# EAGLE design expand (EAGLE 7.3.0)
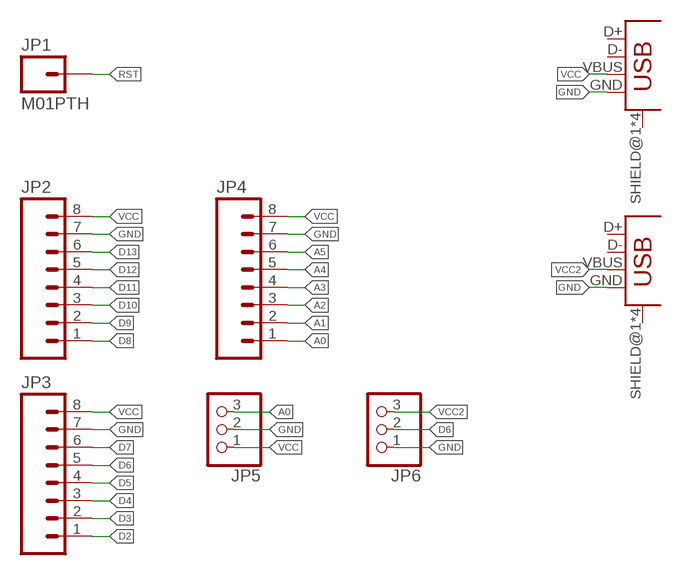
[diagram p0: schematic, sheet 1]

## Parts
JP1  M01PTH  [1X01]
JP2  M08  [1X08]
JP3  M08  [1X08]
JP4  M08  [1X08]
JP5  PINHD-1X3  [1X03]
JP6  PINHD-1X3  [1X03]
U$1  USB_MINIB  [USB_MINIB]
U$2  USB_MINIB  [USB_MINIB]

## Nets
A0: JP4.1 JP5.3
A1: JP4.2
A2: JP4.3
A3: JP4.4
A4: JP4.5
A5: JP4.6
D2: JP3.1
D3: JP3.2
D4: JP3.3
D5: JP3.4
D6: JP3.5 JP6.2
D7: JP3.6
D8: JP2.1
D9: JP2.2
D10: JP2.3
D11: JP2.4
D12: JP2.5
D13: JP2.6
GND: JP2.7 JP3.7 JP4.7 JP5.2 JP6.1 U$1.GND U$2.GND
RST: JP1.1
VCC: JP2.8 JP3.8 JP4.8 JP5.1 U$1.VBUS
VCC2: JP6.3 U$2.VBUS
Unconnected: U$1.D+ U$1.D- U$1.SHIELD@1(SHIELD) U$1.SHIELD@2(SHIELD) U$1.SHIELD@3(SHIELD) U$1.SHIELD@4(SHIELD) U$2.D+ U$2.D- U$2.SHIELD@1(SHIELD) U$2.SHIELD@2(SHIELD) U$2.SHIELD@3(SHIELD) U$2.SHIELD@4(SHIELD)

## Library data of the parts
JP1 = 01_SparkFun:M01: Header 1
JP2-JP4 = 01_SparkFun:M08: Header 8 Standard 8-pin 0.1" header. Use with straight break away headers (SKU : PRT-00116), right angle break away headers (PRT-00553), swiss pins (PRT-00743), machine pins (PRT-00117), and female headers (PRT-00115).
JP5 JP6 = adafruit:PINHD-1X3: PIN HEADER
U$1 U$2 = fab:USB_MINIB

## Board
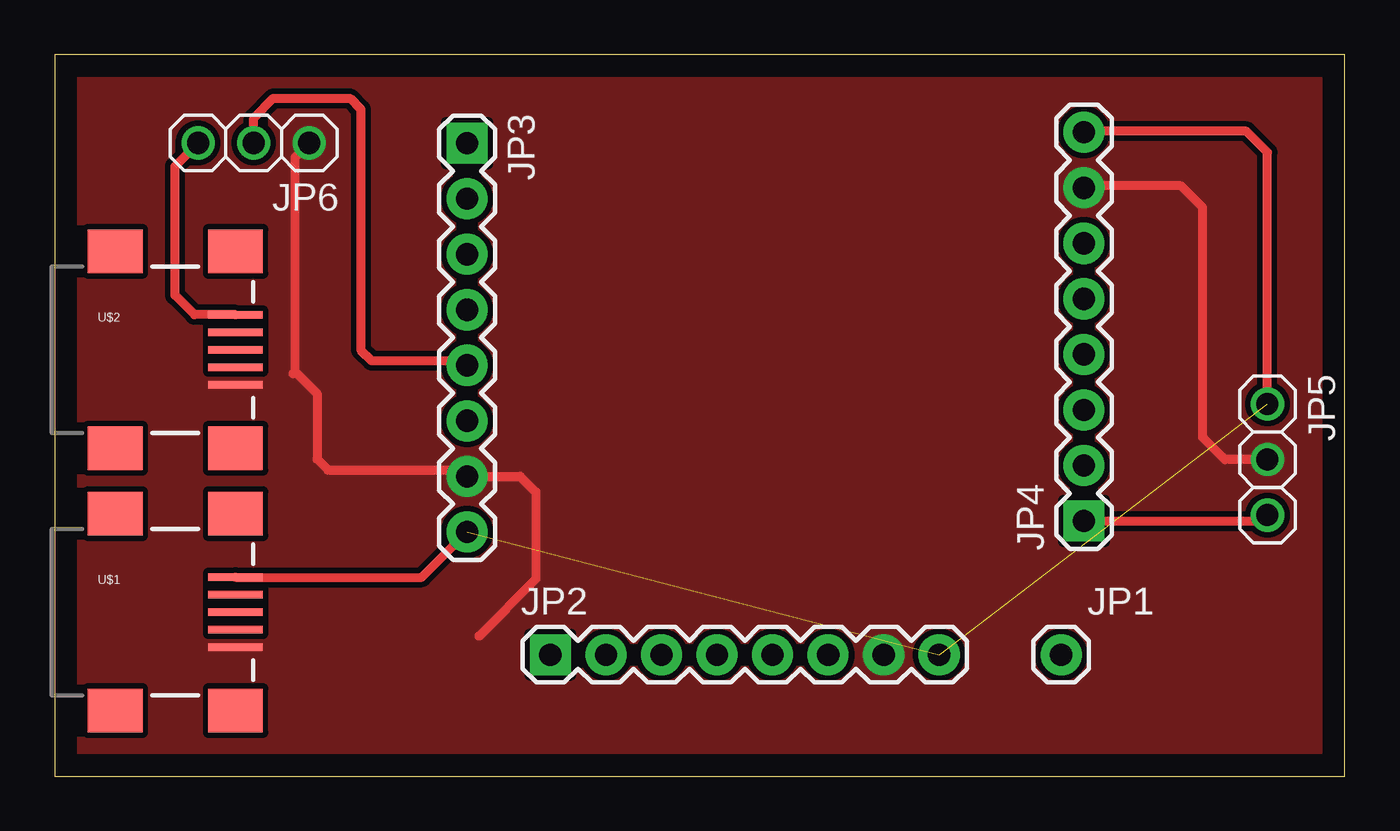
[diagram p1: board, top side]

Size 59 x 33 mm. Coordinates in mm from the lower left corner, seen from the top.
Outline: 0,0 59,0 59,33 0,33 0,0
Copper layers (1*16): Top 0.035mm / dielectric 1.5mm / Bottom 0.035mm
Design rules "default": minimum track width 10mil, minimum drill 24mil, track to track 8mil, track to pad 8mil, pad to pad 8mil, via to via 8mil, smd to smd 8mil, copper to edge 40mil, drill to drill 8mil, minimum pad ring 10mil, minimum via ring 8mil, stop-mask expansion 4mil, vias tented up to drill 0mil, thermal gap 10mil

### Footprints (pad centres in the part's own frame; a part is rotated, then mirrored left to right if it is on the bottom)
1X01 = drill 1.016 pad 1.88: 1 0,0
1X08 = drill 1.016 pad 1.88 square: 1 0,0 | drill 1.016 pad 1.88: 2 2.54,0; 3 5.08,0; 4 7.62,0; 5 10.16,0; 6 12.7,0; 7 15.24,0; 8 17.78,0
1X03 = drill 1.016: 1 -2.54,0; 2 0,0; 3 2.54,0
USB_MINIB = smd 2.5 x 0.35: D+ 3.77,0; D- 3.77,0.8; GND 3.77,-1.6; ID 3.77,-0.8; VBUS 3.77,1.6 | smd 2.5 x 2: SHIELD@1 -1.73,-4.5; SHIELD@2 -1.73,4.5; SHIELD@3 3.77,4.5; SHIELD@4 3.77,-4.5

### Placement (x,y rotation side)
JP1  46.03,5.55 0 top
JP2  22.67,5.55 0 top
JP3  18.86,28.95 270 top
JP4  47.07,11.67 90 top
JP5  55.46,14.48 270 top
JP6  9.1,28.96 180 top
U$1  4.5,7.5 0 top
U$2  4.5,19.5 0 top

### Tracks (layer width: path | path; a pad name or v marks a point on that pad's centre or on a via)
A0
  Top 0.406: JP4.1 55.19,11.67 JP5.3
D6
  Top 0.406: JP6.2 9.1,30.1 10,31 13.5,31 14,30.5 14,19.5 14.5,19 18.65,19 JP3.5
GND
  Top 0.406: JP5.2 53.52,14.48 52.5,15.5 52.5,26 51.5,27 47.16,27 JP4.7 | 19.4,6.4 22,9 22,13 21.29,13.71 JP3.7 18.57,14 12.5,14 12,14.5 12,17.5 11.1,18.4 | 10.9,18.4 11,18.5 11,28.32 JP6.1
  pour Top (isolate 0.254, no thermals): 1,1 58,1 58,32 0.5,32.5
VCC  (2 unrouted)
  Top 0.406: JP5.1 55.46,28.54 54.5,29.5 47.12,29.5 JP4.8 | U$1.VBUS 16.79,9.1 JP3.8
VCC2
  Top 0.406: U$2.VBUS 6.4,21.1 5.5,22 5.5,27.9 JP6.3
